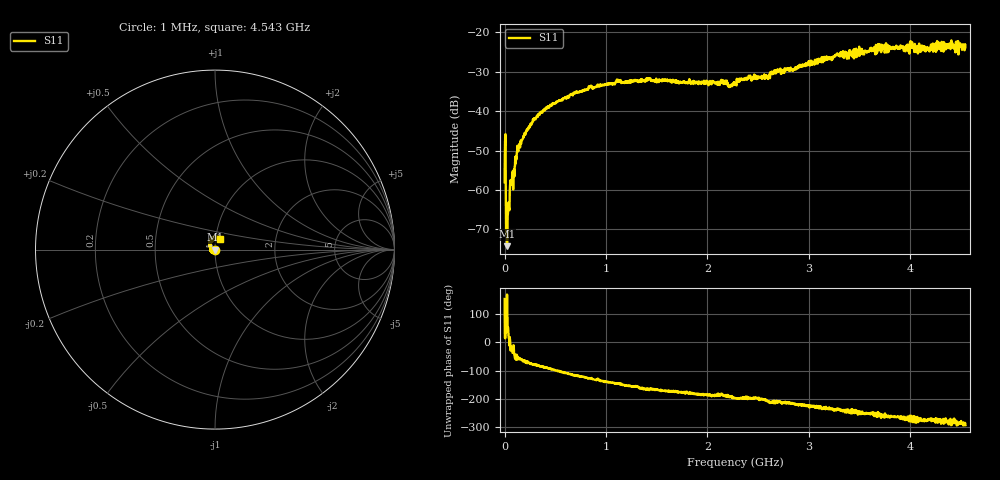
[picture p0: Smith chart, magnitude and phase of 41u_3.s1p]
# HZ S RI R 50
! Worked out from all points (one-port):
!   1515 points, 1 MHz to 4.543 GHz, reference 50 ohm
!   lowest |S11| = -74.2 dB at 25 MHz (marker M1), VSWR 1.00, Z = 50 + j0.00332 ohm
!   |S11| at or under -10 dB: start of sweep to end of sweep
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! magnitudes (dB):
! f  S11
! 1 MHz  -58.0
! 7 MHz  -45.9
! 25 MHz  -74.2
! 34 MHz  -65.9
! 58 MHz  -57.5
! 73 MHz  -58.6
! 124 MHz  -50.3
! 208 MHz  -45.6
! 340 MHz  -40.6
! 571 MHz  -37.3
! 841 MHz  -33.7
! 1.138 GHz  -32.4
! 1.417 GHz  -32.0
! 1.705 GHz  -32.7
! 2.155 GHz  -33.0
! 2.224 GHz  -33.4
! 2.272 GHz  -32.9
! 2.401 GHz  -31.8
! 2.596 GHz  -31.3
! 2.698 GHz  -29.9
! 2.842 GHz  -29.8
! 3.298 GHz  -25.8
! 3.409 GHz  -24.6
! 3.697 GHz  -23.5
! 3.976 GHz  -24.0
! 4.171 GHz  -23.9
! 4.393 GHz  -23.2
! 4.543 GHz  -23.8
